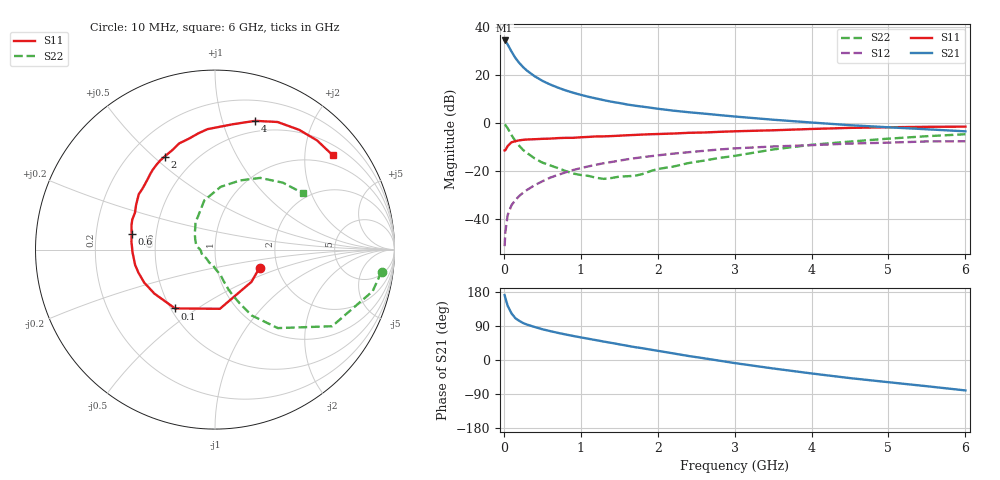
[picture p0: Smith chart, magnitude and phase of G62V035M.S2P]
! SIEMENS Small Signal Semiconductors
! BFG193
! Si NPN RF Bipolar Junction Transistor in SOT223
! VCE = 2 V  IC = 35 mA
! Common Emitter S-Parameters:  August  1996
# GHz  S  MA  R  50
!  f  S11  S21  S12  S22
! GHz  MAG  ANG  MAG  ANG  MAG  ANG  MAG  ANG
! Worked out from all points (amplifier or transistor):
!   36 points, 10 MHz to 6 GHz, reference 50 ohm
!   highest |S21| = 34.4 dB at 10 MHz (marker M1)
!   |S21| within 3 dB of that: start of sweep to 72.06 MHz
!   unconditionally stable (mu >= 1): 464.2 MHz to 2.623 GHz
!   at 250 MHz: K = 0.87, MSG = 26.2 dB, |S12| = -29.1 dB
!   at 1.4 GHz: K = 1.05, MAG = 11.1 dB, |S12| = -16.3 dB
!   at 6 GHz: K = 0.92, MSG = 2.1 dB, |S12| = -7.6 dB
!   S11 on the Smith chart (normalised r, x): 10 MHz: 1.61, -0.35; 100 MHz: 0.53, -0.41; 600 MHz: 0.36, +0.08; 2 GHz: 0.34, +0.54; 4 GHz: 0.39, +1.28; 6 GHz: 0.74, +2.66
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0.01  0.2681 -22.0  52.73 171.3  0.0027 87.9  0.9363 -7.5
0.02  0.2712 -41.5  51.14 163.7  0.0054 82.3  0.9084 -14.8
0.05  0.331 -85.3  43.31 142.8  0.0121 69.2  0.7797 -33.2
0.1  0.3962 -124.2  30.93 122.9  0.0194 63.6  0.5604 -51.3
0.15  0.4173 -144.0  22.78 110.3  0.0247 62.0  0.4199 -60.9
0.2  0.4351 -154.9  17.96 103.3  0.0301 63.7  0.3358 -65.0
0.25  0.4456 -163.3  14.68 97.6  0.0352 64.0  0.2741 -68.7
0.3  0.4532 -169.2  12.41 93.5  0.0401 65.0  0.238 -71.1
0.4  0.4596 -177.9  9.461 87.2  0.0504 65.6  0.183 -74.6
0.5  0.4677 174.5  7.603 81.2  0.0608 65.1  0.1497 -77.2
0.6  0.4726 169.1  6.378 76.4  0.0723 64.3  0.131 -80.8
0.8  0.4903 160.0  4.805 67.5  0.0933 61.2  0.1001 -91.5
1.1  0.5133 147.6  3.525 56.0  0.1247 56.3  0.0789 -114.2
1.6  0.5553 130.4  2.44 37.7  0.1747 45.4  0.0776 -164.2
2  0.5894 118.4  1.987 24.3  0.2115 36.2  0.1098 163.8
2.2  0.6033 113.2  1.814 17.5  0.2297 31.5  0.1231 153.5
2.8  0.6542 98.2  1.464 -1.7  0.2808 17.4  0.1869 125.6
3.5  0.7054 81.9  1.172 -22.3  0.324 -0.1  0.281 102.2
4  0.7514 72.7  1.024 -35.5  0.3453 -9.9  0.3513 84.8
4.5  0.7917 63.9  0.901 -47.8  0.3731 -19.9  0.41 70.0
5.5  0.8328 46.9  0.74 -69.2  0.4132 -42.9  0.5311 44.6
6  0.8403 38.8  0.671 -80.3  0.4166 -56.0  0.5835 32.4
